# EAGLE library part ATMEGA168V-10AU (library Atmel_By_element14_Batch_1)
Microcontroller
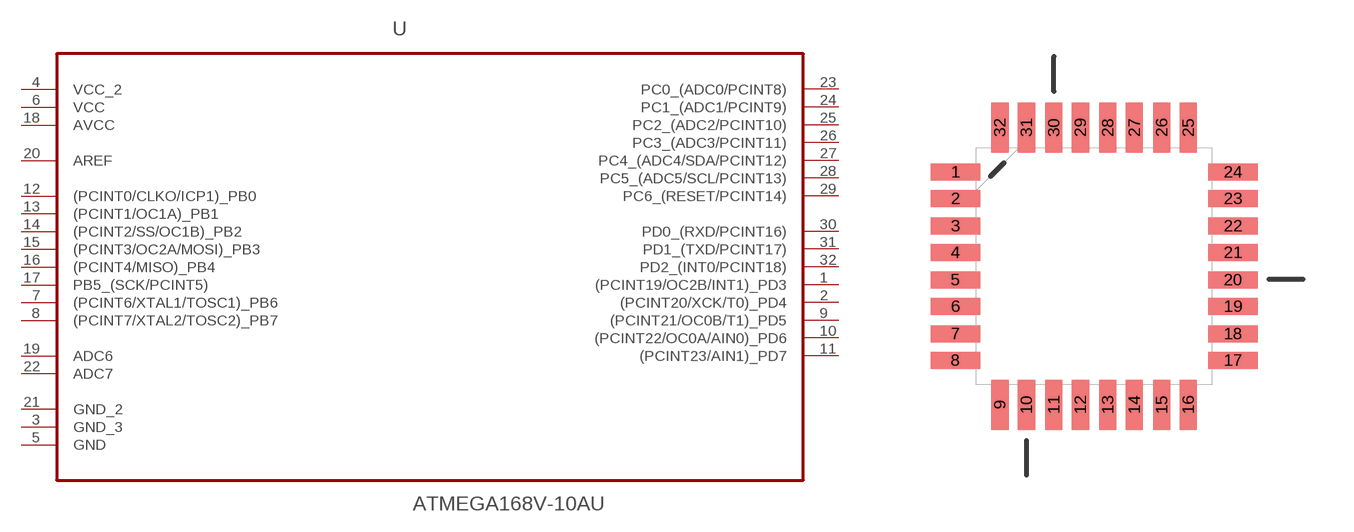
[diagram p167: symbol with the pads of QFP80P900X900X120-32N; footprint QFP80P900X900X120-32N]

Designator prefix U

## ATMEGA168V-10AU (DESCRIPTION: Microcontroller; MPN: ATMEGA168V-10AU; OC_FARNELL: 9171215; OC_NEWARK: 73M8857; PACKAGE: QFP-32; SUPPLIER: ATMEL)  [QFP80P900X900X120-32N]
1  (PCINT19/OC2B/INT1)_PD3
2  (PCINT20/XCK/T0)_PD4
3  GND_3  pas
4  VCC_2  pwr
5  GND  pas
6  VCC  pwr
7  (PCINT6/XTAL1/TOSC1)_PB6
8  (PCINT7/XTAL2/TOSC2)_PB7
9  (PCINT21/OC0B/T1)_PD5
10  (PCINT22/OC0A/AIN0)_PD6
11  (PCINT23/AIN1)_PD7
12  (PCINT0/CLKO/ICP1)_PB0
13  (PCINT1/OC1A)_PB1
14  (PCINT2/SS/OC1B)_PB2
15  (PCINT3/OC2A/MOSI)_PB3
16  (PCINT4/MISO)_PB4
17  PB5_(SCK/PCINT5)
18  AVCC  pwr
19  ADC6  in
20  AREF  in
21  GND_2  pas
22  ADC7  in
23  PC0_(ADC0/PCINT8)
24  PC1_(ADC1/PCINT9)
25  PC2_(ADC2/PCINT10)
26  PC3_(ADC3/PCINT11)
27  PC4_(ADC4/SDA/PCINT12)
28  PC5_(ADC5/SCL/PCINT13)
29  PC6_(RESET/PCINT14)
30  PD0_(RXD/PCINT16)
31  PD1_(TXD/PCINT17)
32  PD2_(INT0/PCINT18)

## Footprint QFP80P900X900X120-32N (pad centres in mm)
smd 1.473 x 0.508: 1 -4.115,2.794; 2 -4.115,2.007; 3 -4.115,1.194; 4 -4.115,0.406; 5 -4.115,-0.406; 6 -4.115,-1.194; 7 -4.115,-2.007; 8 -4.115,-2.794; 17 4.115,-2.794; 18 4.115,-2.007; 19 4.115,-1.194; 20 4.115,-0.406; 21 4.115,0.406; 22 4.115,1.194; 23 4.115,2.007; 24 4.115,2.794
smd 0.508 x 1.473: 9 -2.794,-4.115; 10 -2.007,-4.115; 11 -1.194,-4.115; 12 -0.406,-4.115; 13 0.406,-4.115; 14 1.194,-4.115; 15 2.007,-4.115; 16 2.794,-4.115; 25 2.794,4.115; 26 2.007,4.115; 27 1.194,4.115; 28 0.406,4.115; 29 -0.406,4.115; 30 -1.194,4.115; 31 -2.007,4.115; 32 -2.794,4.115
